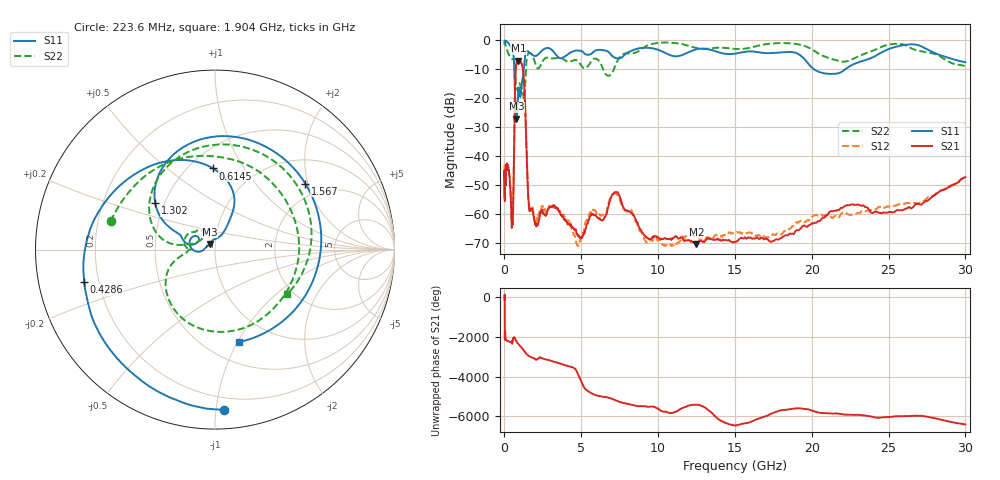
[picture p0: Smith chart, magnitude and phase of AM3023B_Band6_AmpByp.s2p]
# Hz S DB R 50.0
!freq dBS11 angS11 dBS21 angS21 dBS12 angS12 dBS22 angS22
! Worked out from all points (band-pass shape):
!   1601 points, 10 MHz to 30 GHz, reference 50 ohm
!   highest |S21| = -7.23 dB at 903.4 MHz (marker M1); lowest = -70.6 dB at 12.5 GHz (marker M2)
!   |S21| within 3 dB of the highest: 734.2 MHz to 1.202 GHz (467.6 MHz wide, 48.3 % of centre)
!   lowest |S11| = -27.2 dB at 773.6 MHz (marker M3), VSWR 1.09, Z = 47 + j3.03 ohm
!   |S11| at or under -10 dB: 636.6 MHz to 1.26 GHz (623.7 MHz wide, 65.8 % of centre); 20.11 GHz to 22.23 GHz (2.121 GHz wide, 10 % of centre)
!   |S22| runs from -20.6 to -0.9 dB; largest |S21 - S12| = 0.012
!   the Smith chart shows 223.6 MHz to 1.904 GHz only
!   S11 on the Smith chart (normalised r, x): 223.6 MHz: 0.12, -1.05; 428.6 MHz: 0.14, -0.12; 614.5 MHz: 0.65, +0.74; 1.302 GHz: 0.45, +0.28; 1.567 GHz: 1.60, +1.92; 1.904 GHz: 0.71, -1.02
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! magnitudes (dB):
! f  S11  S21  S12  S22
! 10 MHz  -0.4  -45.1  -43.1  -0.9
! 38.04 MHz  -0.2  -50.6  -49.8  -1.2
! 144.7 MHz  -0.6  -43.2  -43.4  -3.2
! 223.6 MHz  -1.0  -43.8  -43.6  -4.4
! 428.6 MHz  -2.5  -56.6  -56.4  -6.3
! 547.7 MHz  -4.2  -61.2  -60.7  -6.7
! 614.5 MHz  -6.9  -44.0  -43.7  -6.9
! 692.9 MHz  -21.3  -15.4  -15.3  -11.1
! 773.6 MHz  -27.2  -8.5  -8.5  -15.9
! 903.4 MHz  -17.3  -7.2  -7.2  -16.7
! 1.302 GHz  -7.5  -17.1  -17.1  -19.4
! 1.567 GHz  -4.1  -55.8  -55.2  -4.7
! 1.904 GHz  -5.5  -61.0  -60.9  -6.5
! 2.084 GHz  -5.5  -64.3  -63.6  -9.3
! 3.141 GHz  -3.8  -57.5  -57.2  -6.4
! 4.805 GHz  -3.7  -67.7  -71.2  -7.5
! 7.1 GHz  -5.9  -53.0  -53.3  -10.5
! 7.926 GHz  -4.7  -58.8  -59.2  -4.6
! 9.349 GHz  -2.8  -68.7  -69.7  -1.8
! 12.5 GHz  -3.3  -70.6  -67.6  -2.8
! 17.92 GHz  -4.4  -68.6  -67.2  -1.1
! 30 GHz  -7.7  -47.4  -47.5  -9.2
